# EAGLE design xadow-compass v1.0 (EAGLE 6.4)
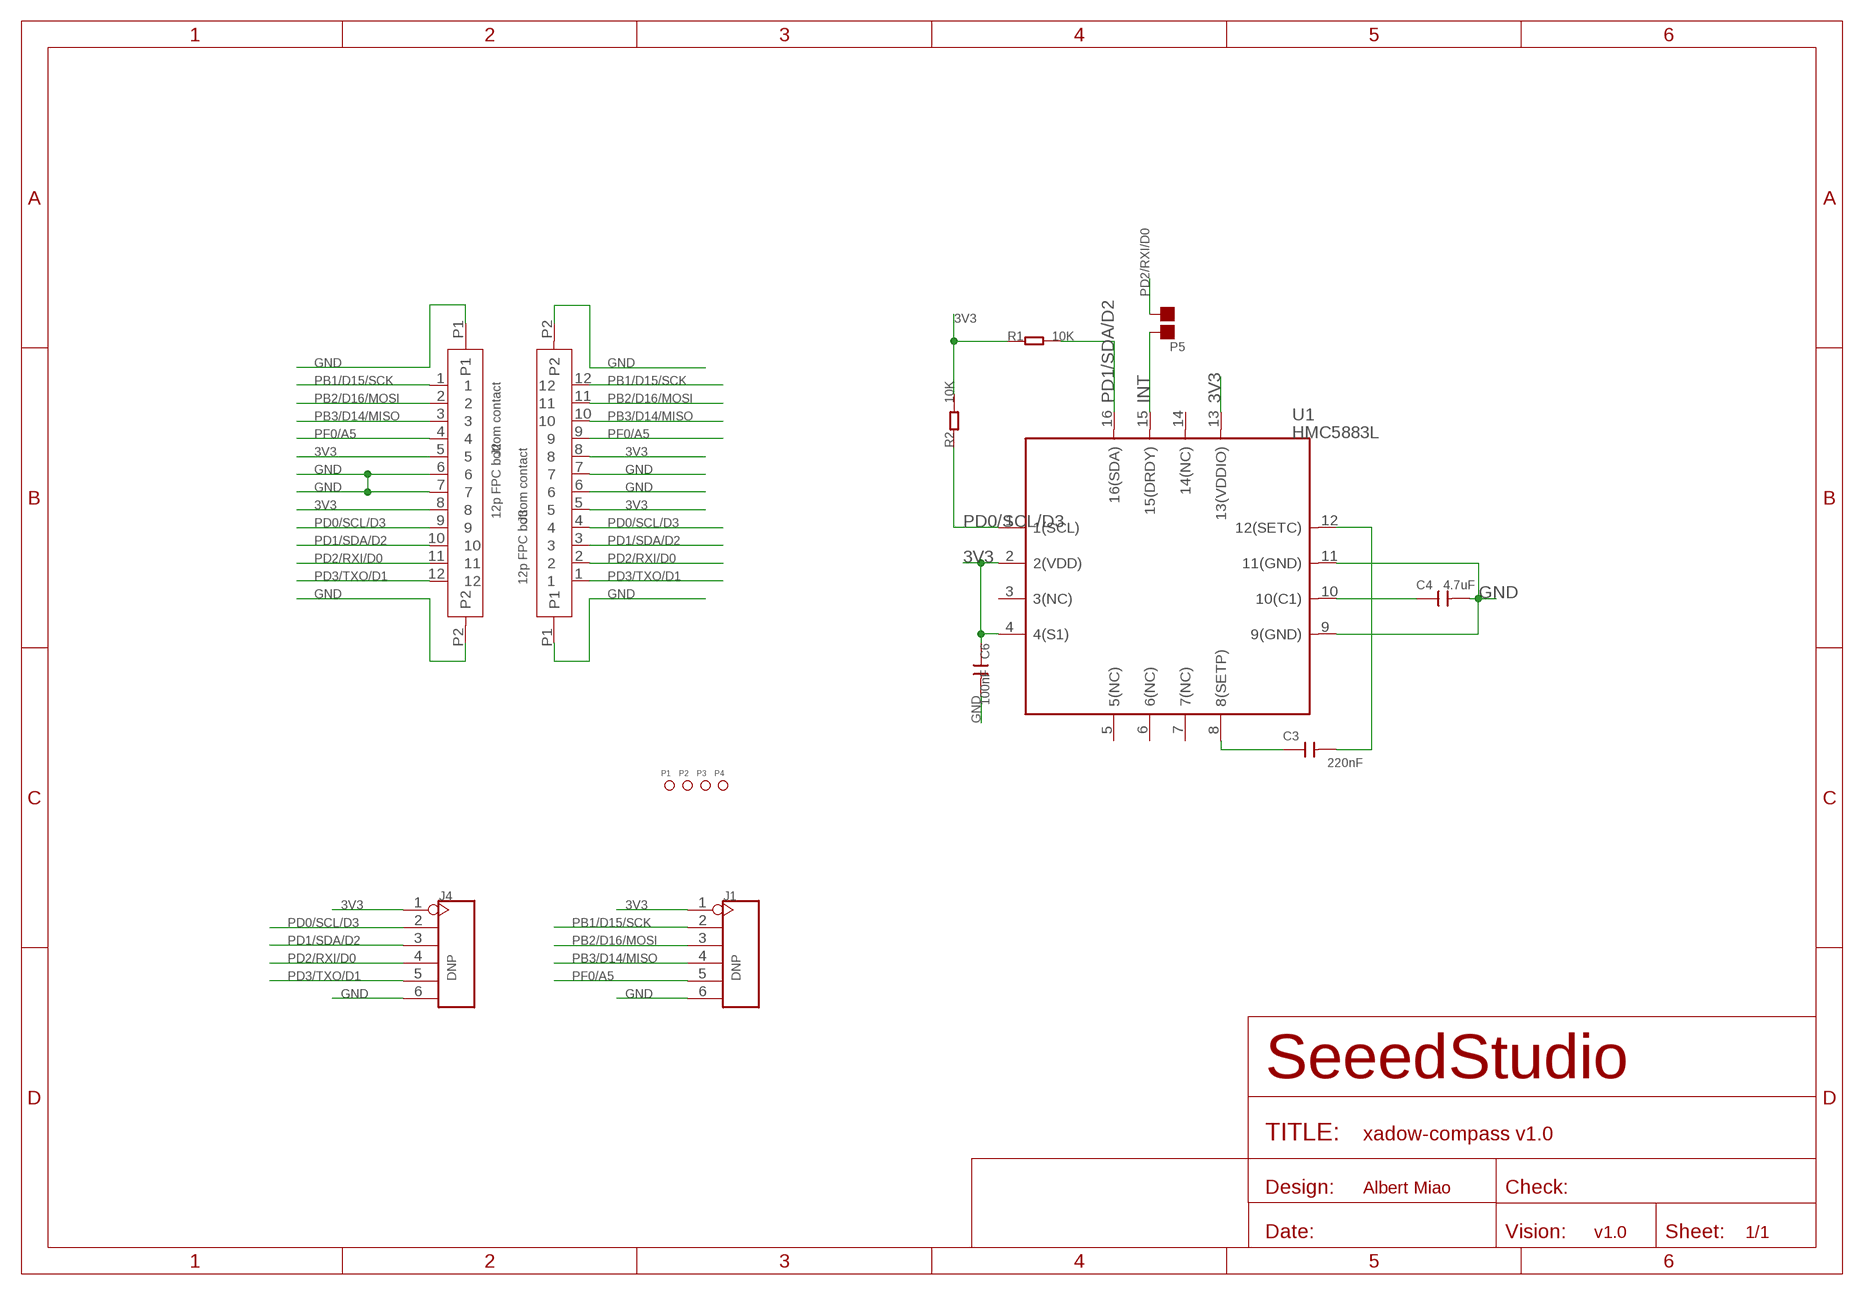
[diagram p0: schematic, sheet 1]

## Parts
C3  220nF  C-0603  [C0603]
C4  4.7uF  C-0805  [C0805]
C6  100nF  C-0603  [C0603]
J1  DNP  HEADER-6P-65/35MIL  [6P-2.54-65/35MIL]
J2  12p FPC bottom contact  FPC052002-12LT  [12P-0.5]
J3  12p FPC bottom contact  FPC052002-12LT  [12P-0.5]
J4  DNP  HEADER-6P-65/35MIL  [6P-2.54-65/35MIL]
P1  PAD-MARK  [ROUND-MARK-1.0]
P2  PAD-MARK  [ROUND-MARK-1.0]
P3  PAD-MARK  [ROUND-MARK-1.0]
P4  PAD-MARK  [ROUND-MARK-1.0]
P5  DNP  PAD-JUMPER-2P  [2P-SMD-1.78X1.27]
R1  10K  R-0603  [R0603]
R2  10K  R-0603  [R0603]
U1  HMC5883L  HMC5883HMC5883  [HMC5883]

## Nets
3V3: C6.1 J1.1 J2.5 J2.8 J3.5 J3.8 J4.1 R1.1 R2.2 U1.2(2(VDD)) U1.4(4(S1)) U1.13(13(VDDIO))
GND: C4.2 C6.2 J1.6 J2.6 J2.7 J2.P1 J2.P2 J3.6 J3.7 J3.P1 J3.P2 J4.6 U1.9(9(GND)) U1.11(11(GND))
INT: P5.2 U1.15(15(DRDY))
N$1: C3.1 U1.8(8(SETP))
N$2: C3.2 U1.12(12(SETC))
N$4: C4.1 U1.10(10(C1))
PB1/D15/SCK: J1.2 J2.1 J3.12
PB2/D16/MOSI: J1.3 J2.2 J3.11
PB3/D14/MISO: J1.4 J2.3 J3.10
PD0/SCL/D3: J2.9 J3.4 J4.2 R2.1 U1.1(1(SCL))
PD1/SDA/D2: J2.10 J3.3 J4.3 R1.2 U1.16(16(SDA))
PD2/RXI/D0: J2.11 J3.2 J4.4 P5.1
PD3/TXO/D1: J2.12 J3.1 J4.5
PF0/A5: J1.5 J2.4 J3.9
Unconnected: U1.3(3(NC)) U1.5(5(NC)) U1.6(6(NC)) U1.7(7(NC)) U1.14(14(NC))

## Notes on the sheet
- Albert Miao
- v1.0

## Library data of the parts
C3 C4 C6 = Discrete:C*: Ceramic Capacitors
J1 J4 = Connector:HEADER-6P
J2 J3 = template:FPC052002-12LT
P1-P4 = Discrete:PAD-MARK; PARTNO: DNP
P5 = Discrete:PAD-JUMPER-2P; PARTNO: DNP
R1 R2 = Discrete:R*
U1 = sensor:HMC5883

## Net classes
0 default: width 0.152 mm, drill 0.152 mm, clearance 0.152 mm
1 GND: width 0.152 mm, drill 0.305 mm, clearance 0.152 mm to class 0, clearance 0.152 mm

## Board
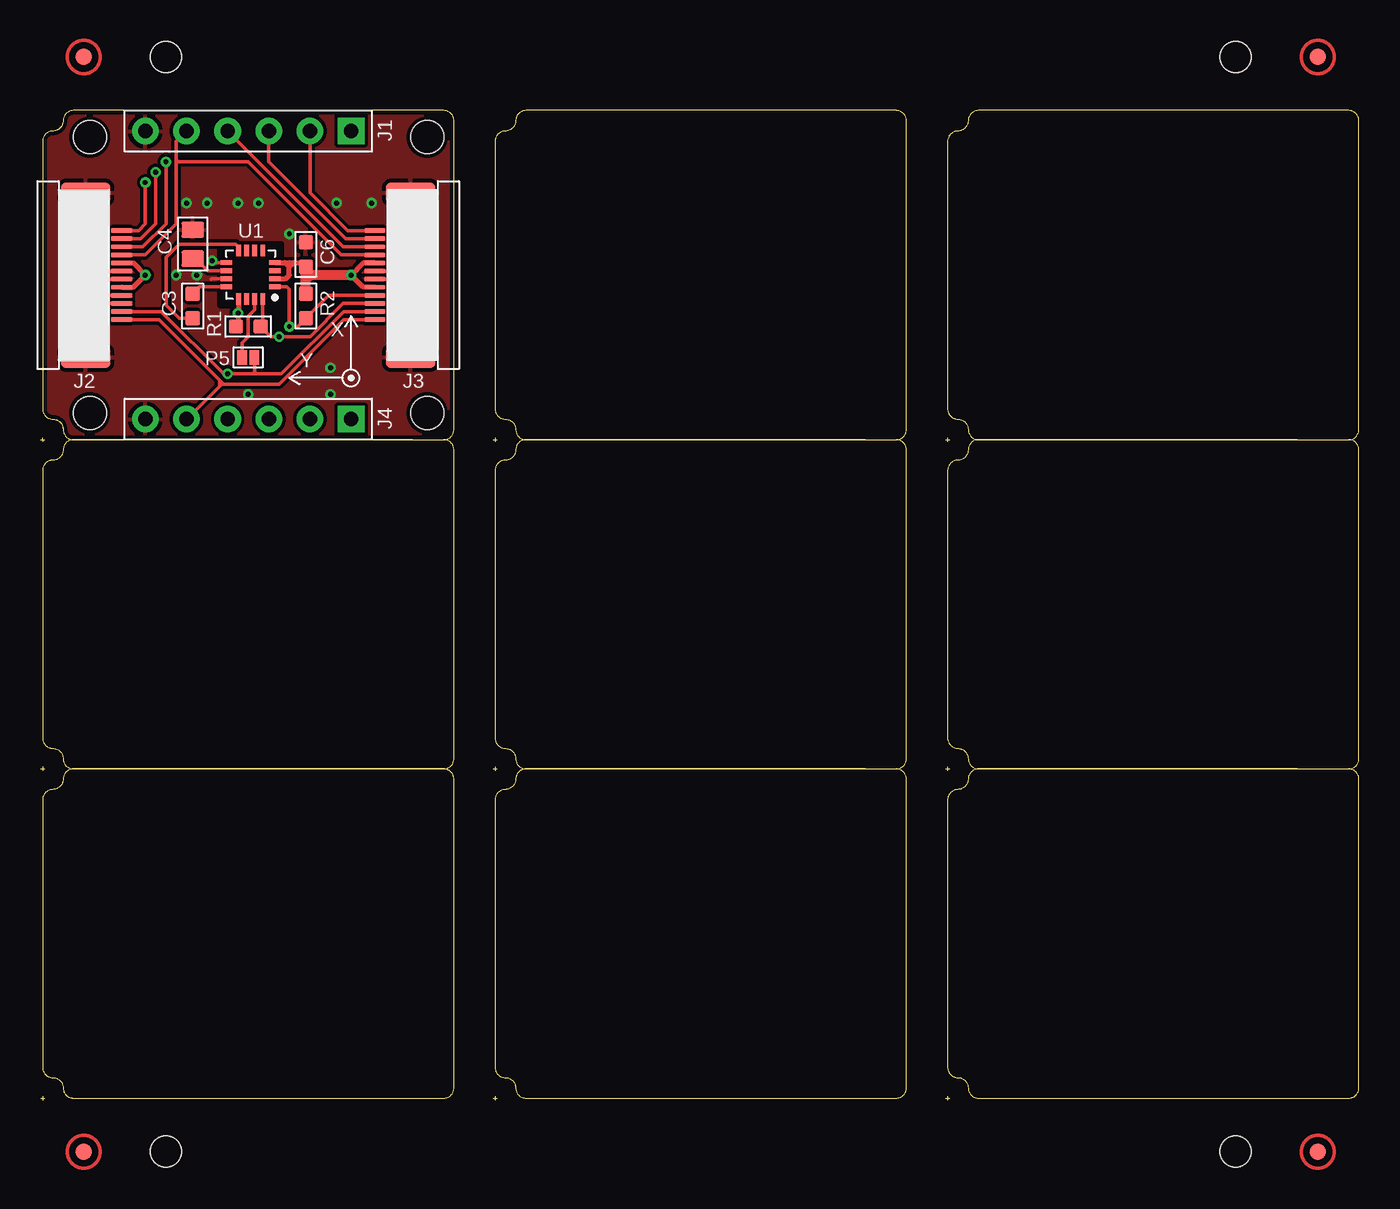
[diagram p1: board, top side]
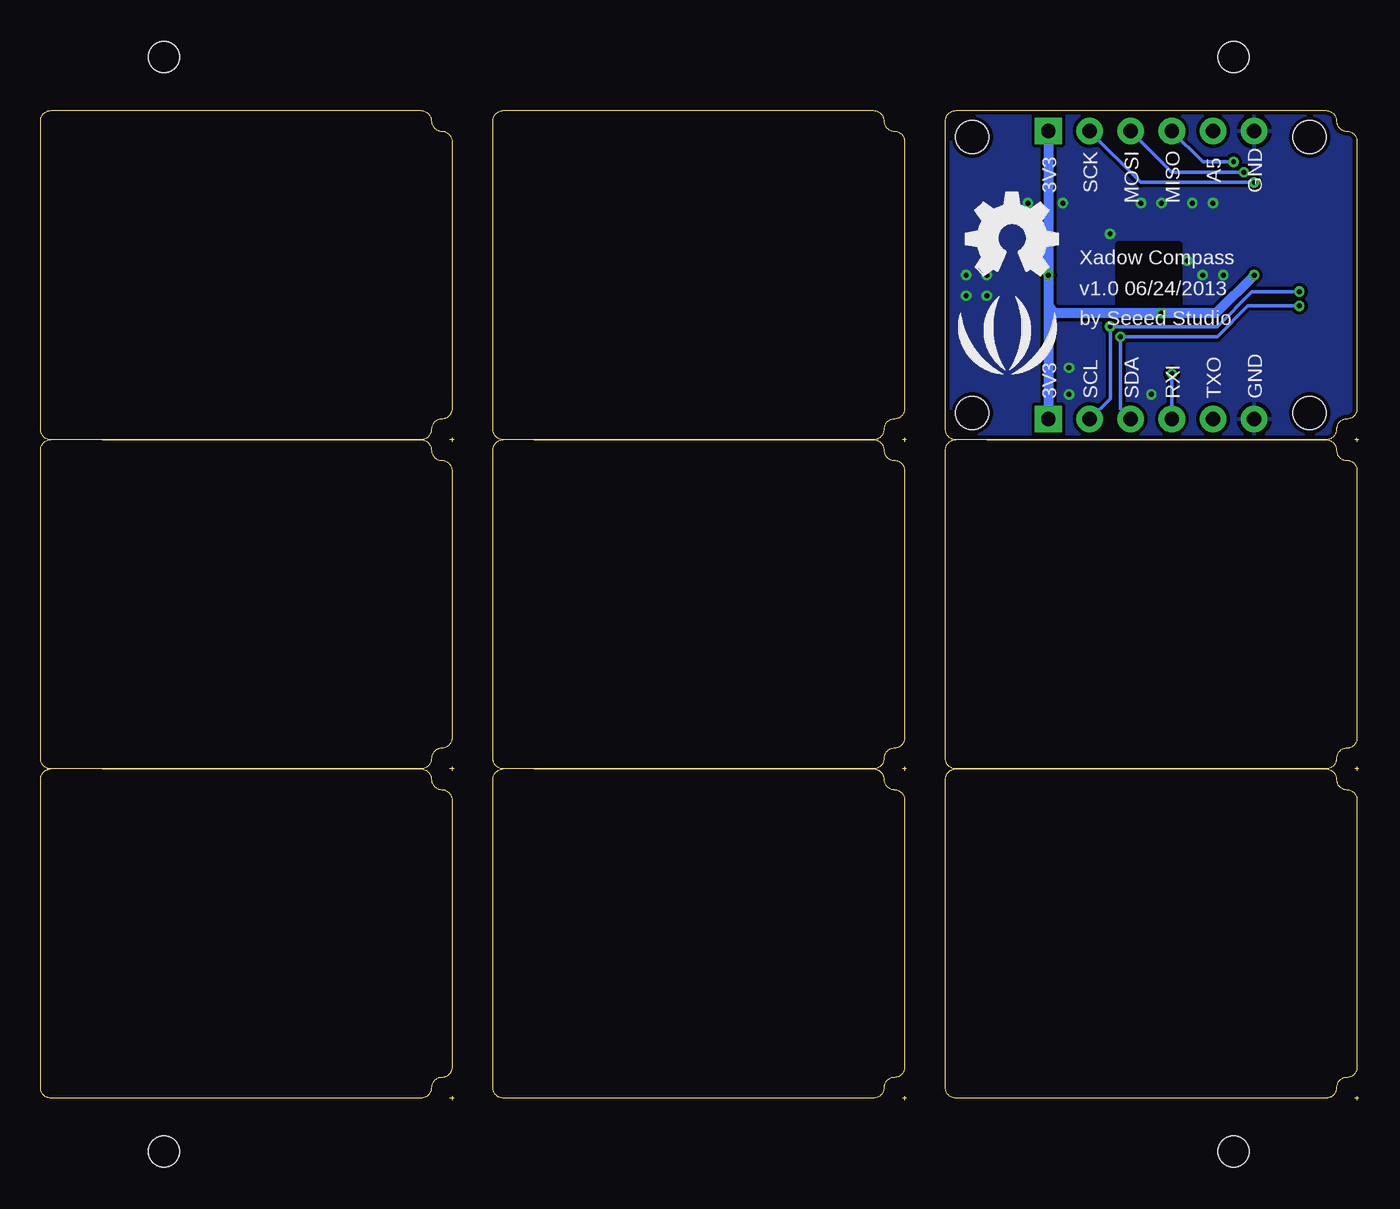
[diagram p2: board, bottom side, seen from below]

Size 81.41 x 61.09 mm. Coordinates in mm from the lower left corner, seen from the top.
Outline: 201 segments
Copper layers (1*16): Top 0.035mm / dielectric 1.5mm / Bottom 0.035mm
Design rules "SeeedStudio_rule_no_angle_090911 *": minimum track width 6mil, minimum drill 12mil, track to track 6mil, track to pad 6mil, pad to pad 6mil, via to via 6mil, smd to smd 0mil, copper to edge 10mil, drill to drill 10mil, minimum pad ring 10mil, minimum via ring 6mil, stop-mask expansion 2mil, vias tented up to drill 100mil, thermal gap 10mil
Holes 2.03 mm at 3.05,42.42 3.05,59.44 23.88,59.44 23.88,42.42
Holes 1.91 mm at 73.79,64.39 7.75,64.39 7.75,-3.17 73.79,-3.17
tRestrict: area 4.6,50.9 to 5.2,51; area 20.4,50.9 to 21,51; area 11.1,49.1 to 14.9,52.8; 13 lines
bRestrict: area 11.1,49.1 to 14.9,52.8; 13 lines

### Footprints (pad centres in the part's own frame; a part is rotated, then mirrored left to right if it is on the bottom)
C0603 = smd 0.889 x 0.889: 1 -0.762,0; 2 0.762,0
C0805 = smd 1.016 x 1.397: 1 -0.889,0; 2 0.889,0
6P-2.54-65/35MIL = drill 0.889 pad 1.651 square: 1 0,6.35 | drill 0.889 pad 1.651: 2 0,3.81; 3 0,1.27; 4 0,-1.27; 5 0,-3.81; 6 0,-6.35
12P-0.5 = smd 0.3 x 1.3: 1 -2.75,2.35; 2 -2.25,2.35; 3 -1.75,2.35; 4 -1.25,2.35; 5 -0.75,2.35; 6 -0.25,2.35; 7 0.25,2.35; 8 0.75,2.35; 9 1.25,2.35; 10 1.75,2.35; 11 2.25,2.35; 12 2.75,2.35 | smd 1.27 x 3.048: P1 -5.08,0.127; P2 5.08,0.127
ROUND-MARK-1.0 = smd 1.016 x 1.016: P$1 0,0
2P-SMD-1.78X1.27 = smd 0.889 x 0.61: 1 0,0.381; 2 0,-0.381
R0603 = smd 0.889 x 0.889: 1 -0.762,0; 2 0.762,0
HMC5883 = smd 0.7 x 0.3: 1 0,2.25; 2 0,1.75; 3 0,1.25; 4 0,0.75; 9 3,0.75; 10 3,1.25; 11 3,1.75; 12 3,2.25 | smd 0.3 x 0.7: 5 0.75,0; 6 1.25,0; 7 1.75,0; 8 2.25,0; 13 2.25,3; 14 1.75,3; 15 1.25,3; 16 0.75,3

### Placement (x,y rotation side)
C3  9.4,49.02 90 top
C4  9.4,52.83 90 top
C6  16.38,52.2 90 top
J1  12.83,59.82 270 top
J2  2.67,50.93 270 top
J3  22.99,50.93 90 top
J4  12.83,42.04 270 top
P1  not placed on the board
P2  not placed on the board
P3  not placed on the board
P4  not placed on the board
P5  12.83,45.85 270 top
R1  12.83,47.75 0 top
R2  16.38,49.02 90 top
U1  14.48,52.45 180 top
U$2  [LOGO_SILK]  21.72,46.48 0 bottom
U$3  [OSHW_FILLX200_NOTEXT]  24.26,50.93 0 bottom

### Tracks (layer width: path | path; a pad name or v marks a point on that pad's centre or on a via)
3V3  (via drill 0.3 pad 0.64)
  Top 0.305: 12.23,47.91 R1.1 | U1.4 15.1,51.7 | 15.1,51.7 15.37,51.7 | 15.37,51.7 16.37,51.7 16.38,51.69 C6.1 | U1.2 15.14,50.7 15.37,50.93 15.37,51.44 | 15.37,51.44 15.37,51.7 | 15.1,51.7 15.37,51.44 | 15.37,51.44 15.62,51.69 | J3.8 19.93,51.68 v19.18,50.93 19.93,50.18 J3.5 | J2.5 5.73,51.68 v6.48,50.93 5.73,50.18 J2.8 | 12.23,47.91 12.23,47.66 12.19,47.62 | U1.13 12.23,48.61 v12.19,48.58 12.23,48.54 12.23,47.91
  Top 0.61: R2.2 16.38,50.67 | 16.38,50.67 16.38,50.93 | 16.38,50.93 C6.1 | v19.18,50.93 17.14,50.93 16.64,50.93 | 16.64,50.93 16.38,50.93 | 16.64,50.93 16.38,50.67
  Bottom 0.61: J1.1 v19.18,50.93 19.18,49.02 | v6.48,50.93 8.83,48.58 v12.19,48.58 18.73,48.58 | 18.73,48.58 19.11,48.58 19.18,48.64 | 19.18,49.02 19.18,48.64 | 19.18,48.64 J4.1 | 18.73,48.58 19.05,48.89 | 18.73,48.58 19.05,48.26 19.05,48.89 | 19.05,48.89 19.18,49.02
GND  (via drill 0.3 pad 0.64)
  Top 0.203: U1.11 10.57,50.7 10.54,50.67 | J2.6 3.81,51.18 | J2.7 3.81,50.68 3.81,50.67 | J3.7 21.84,51.18 | J3.6 21.84,50.68 21.84,50.67 | U1.9 10.72,51.7 v10.6,51.82
  other vias: 10.29,55.37 9.02,55.37 15.37,53.47 24.26,50.93 22.99,49.66 24.26,49.66 17.91,45.21 17.91,43.56 18.29,55.37 22.99,50.93 8.38,50.93 9.65,50.93 12.19,55.37 13.46,55.37 20.45,55.37 12.83,43.56
  pour Top (isolate 0.203): 0.13,40.77 25.53,40.77 25.53,61.09 0.13,61.09 0.13,40.89
  pour Bottom (isolate 0.203): 0.13,40.77 25.53,40.77 25.53,61.09 0.13,61.09 0.13,40.89
INT
  Top 0.203: U1.15 13.23,48.79 12.83,48.39 12.83,47.12 12.45,46.74 P5.2
N$1
  Top 0.203: U1.8 12.23,52.67 12.06,52.83 8.56,52.83 7.75,52.02 7.75,49.07 8.56,48.26 C3.1
N$2
  Top 0.203: U1.12 9.81,50.2 C3.2
N$4
  Top 0.203: U1.10 10.33,51.2 9.84,51.69 9.65,51.69 C4.1
PB1/D15/SCK  (via drill 0.3 pad 0.64)
  Top 0.203: J3.12 18.97,53.68 16.64,56.01 J1.2 | J2.1 6.05,53.68 6.48,54.1 v6.48,56.64
  Bottom 0.203: v6.48,56.64 13.46,56.64 J1.2
PB2/D16/MOSI  (via drill 0.3 pad 0.64)
  Top 0.203: J3.11 18.83,53.18 14.1,57.91 J1.3 | J2.2 6.19,53.18 7.11,54.1 v7.11,57.28
  Bottom 0.203: v7.11,57.28 11.56,57.28 J1.3
PB3/D14/MISO  (via drill 0.3 pad 0.64)
  Top 0.203: J3.10 18.7,52.68 J1.4 | J2.3 6.32,52.68 7.75,54.1 v7.75,57.91
  Bottom 0.203: v7.75,57.91 9.65,57.91 J1.4
PD0/SCL/D3  (via drill 0.3 pad 0.64)
  Top 0.203: J3.4 17.8,49.68 R2.1 | 16.26,48.01 16.38,48.13 R2.1 | U1.1 15.2,50.2 15.37,50.04 v15.37,47.75 15.88,47.75 R2.1 | J2.9 3.92,49.68 v3.68,49.91
  Bottom 0.203: J4.2 15.37,43.31 v15.37,47.75 8.76,47.75 6.6,49.91 v3.68,49.91
PD1/SDA/D2  (via drill 0.3 pad 0.64)
  Top 0.203: U1.16 13.73,47.89 R1.2 | J3.3 18.7,49.18 16.64,47.12 v14.73,47.12 14.22,47.12 R1.2 | 13.91,47.43 R1.2 | J2.10 3.84,49.18 v3.68,49.02
  Bottom 0.203: J4.3 14.73,42.67 v14.73,47.12 8.76,47.12 6.86,49.02 v3.68,49.02
PD2/RXI/D0  (via drill 0.3 pad 0.64)
  Top 0.203: J3.2 18.7,48.68 14.86,44.83 13.34,44.83 | 13.21,44.83 13.08,44.83 | 13.08,44.83 v11.56,44.83 11.3,44.83 7.46,48.68 J2.11 | P5.1 13.21,44.96 | 13.21,44.96 13.21,44.83 | 13.21,44.96 13.34,44.83 | 13.21,44.96 13.08,44.83 | 13.34,44.83 13.21,44.83
  Bottom 0.203: J4.4 v11.56,44.83
PD3/TXO/D1
  Top 0.203: J3.1 18.71,48.18 14.73,44.2 11.3,44.2 | 11.3,44.2 11.24,44.26 | 11.24,44.26 11.05,44.45 | 11.05,44.45 7.32,48.18 J2.12 | J4.5 11.05,44.07 | 11.05,44.07 11.18,44.2 | 11.18,44.2 11.24,44.26 | 11.3,44.2 11.18,44.2 | 11.05,44.07 11.05,44.45
PF0/A5
  Top 0.203: J3.9 18.56,52.18 12.83,57.91 8.51,57.91 | J2.4 6.46,52.18 8.38,54.1 8.38,57.78 | 8.38,57.78 8.38,57.91 | 8.38,57.91 8.38,58.04 | 8.38,58.04 8.38,58.29 8.38,59.18 J1.5 | 8.51,57.91 8.38,57.91 | 8.38,58.04 8.51,57.91 | 8.51,57.91 8.38,57.78 | 8.38,57.91 8.38,58.04

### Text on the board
tPlace: X | Y
bPlace: A5 | GND | SCK | 3V3 | MISO | MOSI | Xadow Compass | v1.0 06/24/2013 | by Seeed Studio | GND | TXO | RXI | SDA | SCL | 3V3
tEnhance: Top Enhance 0.25~0.28mm
bEnhance: Bottom Enhance
bEnHoles: Holes on Bottom Enhance | All Holes are 70mil diameter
